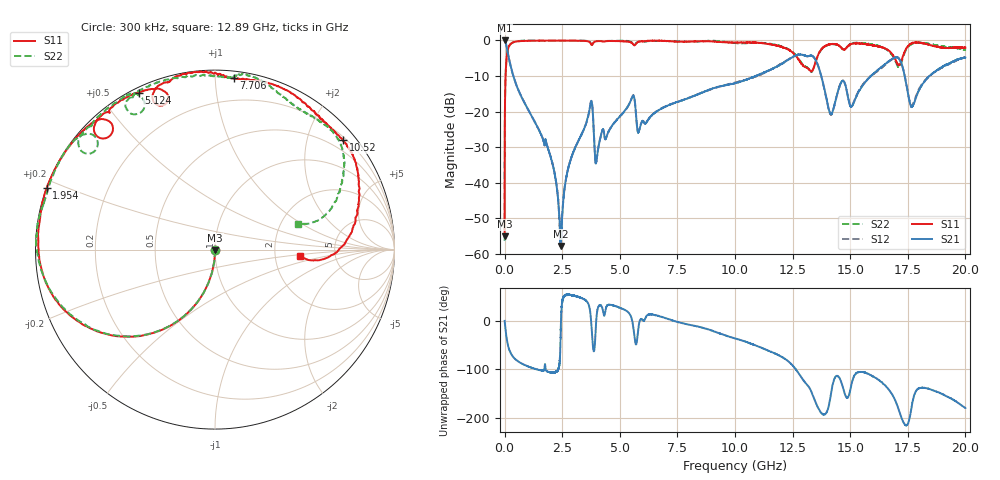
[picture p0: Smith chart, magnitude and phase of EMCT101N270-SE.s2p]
!EMCT101N270
!Johanson Technology Inc.
!www.johansontechnology.com
!Test Board Conditions:
!Substrate Type  RO4350B
!Substrate Thickness  10 mil
!Substrate Dk  3.66
!TL Type: GCPW
!TL Trace Width  22 mil
!TL Gap  14 mil
!PART MODE SINGLE ENDED (AKA BYPASS)
!DUT TOPOLOGY	SERIES-SHUNT
# MHz S  dB  R 50
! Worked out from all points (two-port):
!   20001 points, 300 kHz to 20 GHz, reference 50 ohm
!   highest |S21| = 0.00 dB at 2.3 MHz (marker M1); lowest = -57.8 dB at 2.429 GHz (marker M2)
!   |S21| within 3 dB of the highest: start of sweep to 123.7 MHz
!   lowest |S11| = -55.0 dB at 300 kHz (marker M3), VSWR 1.00, Z = 50.1 - j0.157 ohm
!   |S11| at or under -10 dB: start of sweep to 42 MHz
!   |S22| runs from -56.3 to 0.0 dB; largest |S21 - S12| = 0.021
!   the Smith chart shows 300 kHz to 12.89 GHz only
!   S11 on the Smith chart (normalised r, x): 300 kHz: 1.00, -0.00; 1.954 GHz: 0.00, +0.18; 5.124 GHz: 0.02, +0.63; 7.706 GHz: 0.04, +1.12; 10.52 GHz: 0.26, +2.68; 12.89 GHz: 2.74, -0.24
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0.3  -55.02 -61.8  -0.01 -0.2  0.00 -0.2  -56.30 -50.5
2.3  -34.80 -88.7  -0.00 -1.1  -0.00 -1.1  -34.86 -88.9
103.298  -3.98 -130.7  -2.29 -40.4  -2.27 -40.3  -4.01 -130.6
200.297  -1.54 -149.4  -5.42 -59.0  -5.40 -59.0  -1.59 -149.8
1954.271  -0.01 160.0  -31.81 -106.0  -31.72 -105.8  -0.10 162.8
2429.264  -0.02 151.8  -57.80 -35.9  -56.38 -36.5  -0.08 156.8
2757.259  -0.04 146.2  -35.96 53.2  -36.08 53.3  -0.04 152.4
3334.25  -0.10 137.1  -26.45 47.0  -26.46 47.0  -0.03 144.3
3747.244  -0.95 129.6  -17.20 3.6  -17.18 3.7  -0.89 136.9
4000.24  -0.21 132.2  -33.17 13.0  -33.13 13.0  -0.17 139.7
5124.223  -0.24 116.0  -20.48 24.5  -20.53 24.8  -0.07 120.3
6667.2  -0.06 94.9  -19.68 10.1  -19.64 9.8  -0.13 109.6
7706.184  -0.34 83.7  -16.80 -4.9  -16.82 -4.5  -0.28 89.7
10000.15  -0.58 47.4  -12.01 -36.4  -11.85 -36.4  -0.68 63.1
10520.14  -0.55 40.6  -10.91 -43.9  -10.94 -45.1  -0.73 54.2
12887.11  -6.57 -4.1  -3.99 -116.9  -3.99 -117.2  -6.31 17.5
13334.1  -8.64 22.9  -4.29 -148.2  -4.30 -148.3  -8.75 43.6
14167.09  -1.03 14.0  -20.69 -150.1  -20.83 -150.3  -1.06 30.9
16667.05  -2.81 -50.5  -5.89 -141.2  -6.00 -139.7  -2.97 -24.0
17108.04  -6.95 -38.5  -5.05 176.7  -5.02 177.8  -7.51 -12.4
17686.03  -0.77 -31.7  -18.64 -171.7  -18.40 -171.2  -0.99 -10.1
20000  -2.03 -101.6  -4.81 -179.7  -4.74 -177.8  -2.63 -67.0
